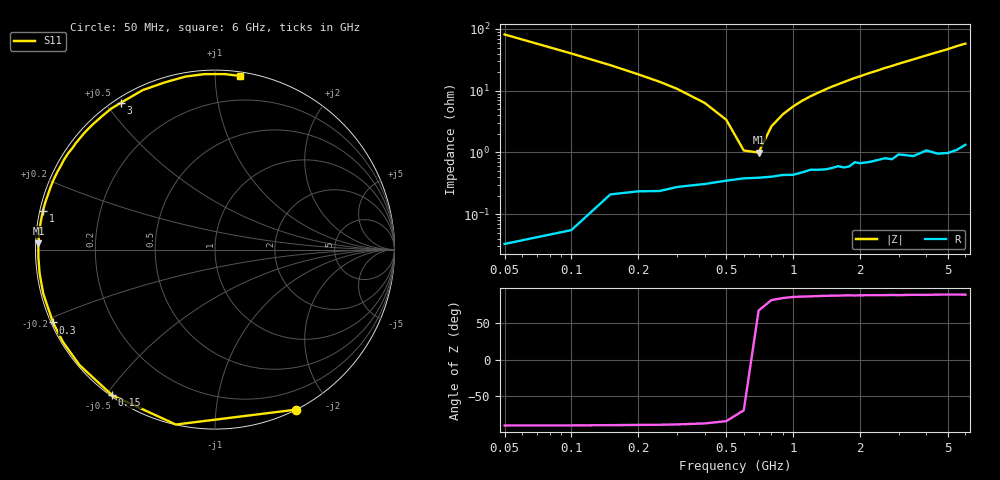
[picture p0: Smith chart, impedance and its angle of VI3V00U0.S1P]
! Infineon Technologies  Discrete & RF Semiconductors
! BB 804
! Si Tuning Diode in SOT23
! VR = 3 V
! S-Parameters:  July  1999
# GHz  S  MA  R  50
!  f  S11
! GHz  MAG  ANG
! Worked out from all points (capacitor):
!   34 points, 50 MHz to 6 GHz, reference 50 ohm
!   read as one part to ground: C = 38.8 pF near 50 MHz
!   lowest |Z| = 995 mohm at 700 MHz (marker M1)
!   series resonance near 652.3 MHz, so ESL is about 1.5 nH
!   S11 on the Smith chart (normalised r, x): 50 MHz: 0.00, -1.63; 150 MHz: 0.00, -0.52; 300 MHz: 0.01, -0.21; 1 GHz: 0.01, +0.11; 3 GHz: 0.02, +0.55; 6 GHz: 0.03, +1.16
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0.05  0.9996 -63.1
0.1  0.9987 -102.6
0.15  0.9935 -125.2
0.2  0.9918 -139.5
0.25  0.9913 -148.8
0.3  0.9895 -155.8
0.4  0.988 -165.6
0.5  0.9862 -172.3
0.6  0.9849 -177.7
0.7  0.9846 177.9
0.8  0.984 174.0
1  0.983 167.4
1.2  0.9798 161.6
1.5  0.979 153.8
1.6  0.9778 151.5
1.8  0.9784 146.7
1.9  0.9752 144.4
2.2  0.976 138.0
2.4  0.9749 134.2
2.6  0.9739 130.0
2.8  0.9756 126.5
3  0.9718 122.7
3.5  0.9757 114.4
4  0.9727 106.6
4.5  0.978 99.6
5  0.9795 93.4
5.5  0.9794 86.8
6  0.9775 81.7
